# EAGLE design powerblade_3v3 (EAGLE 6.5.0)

## Sheet 1 of 6: AC-DC Power Supply
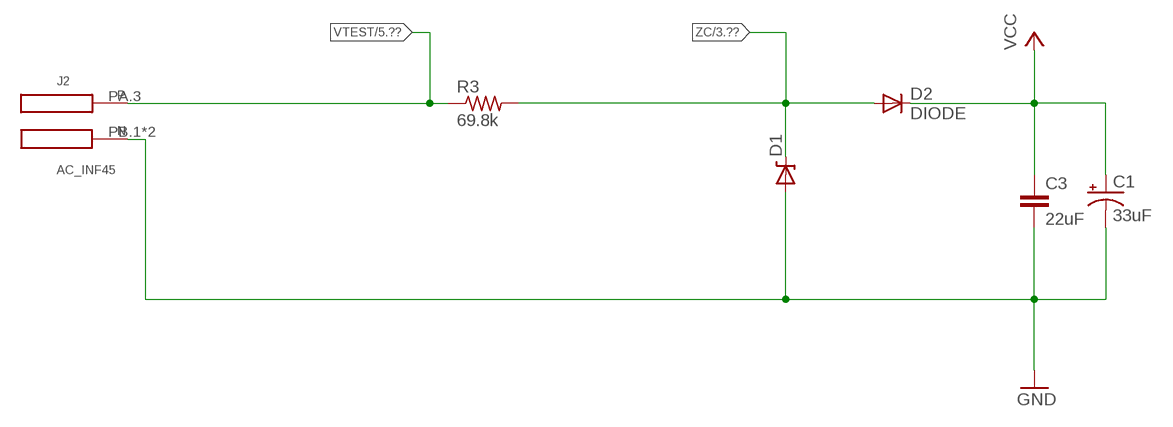
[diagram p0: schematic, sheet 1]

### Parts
C1  33uF  CPOL-US0805_SM  [CPOL0805_SM]
C3  22uF  C-EUC0603_SM  [C0603_SM]
D1  ZENERBZT52  [BZT52]
D2  DIODE  [BAS521]
J2  AC_INF45  [AC3_F45]
R3  69.8k  R-US_R1210  [R1210]

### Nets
GND: C1.- C3.2 D1.A J2.PB.1(N) J2.PB.3(N) ; also sheet 2,3,4,5,6
VCC: C1.+ C3.1 D2.C ; also sheet 2,3,6
VTEST: J2.PA.3(P) R3.1 ; also sheet 5
ZC: D1.C D2.A R3.2 ; also sheet 3,6

## Sheet 2 of 6: Load Supply Regulation
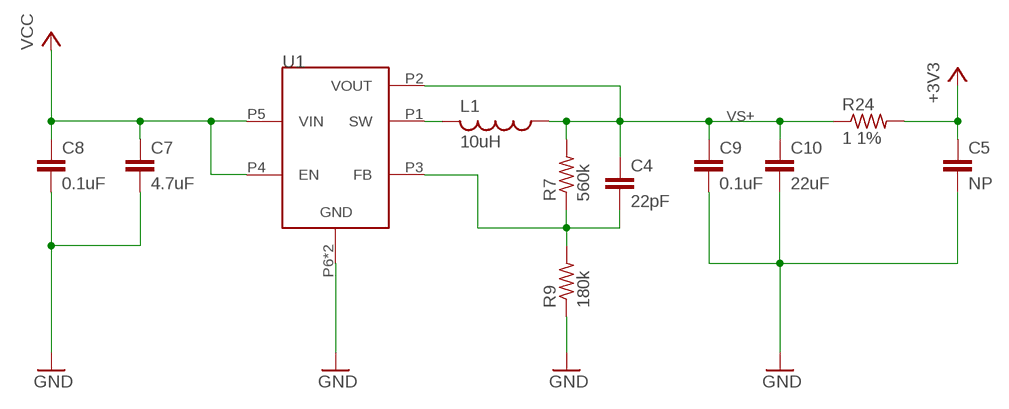
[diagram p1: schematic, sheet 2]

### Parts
C4  22pF  C-EUC0402  [C0402]
C5  NP  C-EUC0603_TN  [C0603_TN]
C7  4.7uF  C-EUC0402  [C0402]
C8  0.1uF  C-EUC0402  [C0402]
C9  0.1uF  C-EUC0402_SM  [C0402_SM]
C10  22uF  C-EUC0603_SM  [C0603_SM]
L1  10uH  L-USL0805  [L0805]
R7  560k  R-US_R0402  [R0402]
R9  180k  R-US_R0402  [R0402]
R24  1 1%  R-US_R0603_SM  [R0603_SM]
U1  TPS62122  [WDFN-6]

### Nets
+3V3: C5.1 R24.2 ; also sheet 3,4,5,6
GND: C5.2 C7.2 C8.2 C9.2 C10.2 R9.1 U1.P6(GND) U1.PAD(GND) ; also sheet 1,3,4,5,6
N$9: L1.2 U1.P1(SW)
N$13: C4.2 R7.1 R9.2 U1.P3(FB)
VCC: C7.1 C8.1 U1.P4(EN) U1.P5(VIN) ; also sheet 1,3,6
VS+: C4.1 C9.1 C10.1 L1.1 R7.2 R24.1 U1.P2(VOUT) ; also sheet 6

## Sheet 3 of 6: MSP430FR5738
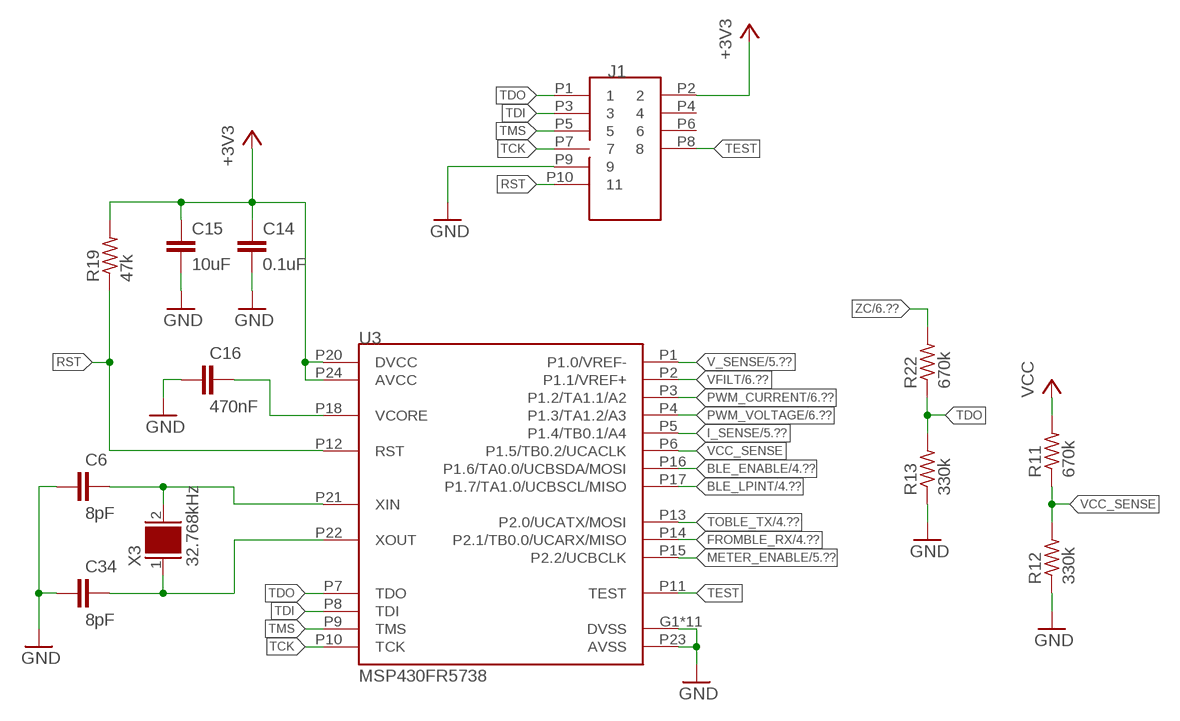
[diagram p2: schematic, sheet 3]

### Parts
C6  8pF  C-EUC0402  [C0402]
C14  0.1uF  C-EUC0402  [C0402]
C15  10uF  C-EUC0603_SM  [C0603_SM]
C16  470nF  C-EUC0402  [C0402]
C34  8pF  C-EUC0402  [C0402]
J1  JTAG_14PIN_IDC-ND  [TC2050-IDC-NL-430-ND]
R11  670k  R-US_R0402  [R0402]
R12  330k  R-US_R0402  [R0402]
R13  330k  R-US_R0402  [R0402]
R19  47k  R-US_R0402  [R0402]
R22  670k  R-US_R0402  [R0402]
U3  MSP430FR5738  [VQFN-24]
X3  32.768kHz  CRYSTAL_0805  [0805]

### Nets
+3V3: C14.1 C15.1 J1.P2 R19.2 U3.P20(DVCC) U3.P24(AVCC) ; also sheet 2,4,5,6
BLE_ENABLE: U3.P16(P1.6/TA0.0/UCBSDA/MOSI) ; also sheet 4
BLE_LPINT: U3.P17(P1.7/TA1.0/UCBSCL/MISO) ; also sheet 4
FROMBLE_RX: U3.P14(P2.1/TB0.0/UCARX/MISO) ; also sheet 4,6
GND: C6.1 C14.2 C15.2 C16.1 C34.1 J1.P9 R12.1 R13.1 U3.G1(DVSS) U3.G2(DVSS) U3.G3(DVSS) U3.G4(DVSS) U3.G5(DVSS) U3.G6(DVSS) U3.G7(DVSS) U3.G8(DVSS) U3.G9(DVSS) U3.P19(DVSS) U3.P23(AVSS) U3.PAD(DVSS) ; also sheet 1,2,4,5,6
I_SENSE: U3.P5(P1.4/TB0.1/A4) ; also sheet 5,6
METER_ENABLE: U3.P15(P2.2/UCBCLK) ; also sheet 5
N$3: C34.2 U3.P22(XOUT) X3.1
N$23: C16.2 U3.P18(VCORE)
N$56: C6.2 U3.P21(XIN) X3.2
PWM_CURRENT: U3.P3(P1.2/TA1.1/A2) ; also sheet 6
PWM_VOLTAGE: U3.P4(P1.3/TA1.2/A3) ; also sheet 6
RST: J1.P10 R19.1 U3.P12(RST)
TCK: J1.P7 U3.P10(TCK)
TDI: J1.P3 U3.P8(TDI)
TDO: J1.P1 R13.2 R22.1 U3.P7(TDO)
TEST: J1.P8 U3.P11(TEST)
TMS: J1.P5 U3.P9(TMS)
TOBLE_TX: U3.P13(P2.0/UCATX/MOSI) ; also sheet 4,6
V_SENSE: U3.P1(P1.0/VREF-) ; also sheet 5,6
VCC: R11.2 ; also sheet 1,2,6
VCC_SENSE: R11.1 R12.2 U3.P6(P1.5/TB0.2/UCACLK)
VFILT: U3.P2(P1.1/VREF+) ; also sheet 5,6
ZC: R22.2 ; also sheet 1,6
Unconnected: J1.P4 J1.P6

## Sheet 4 of 6: nr51822
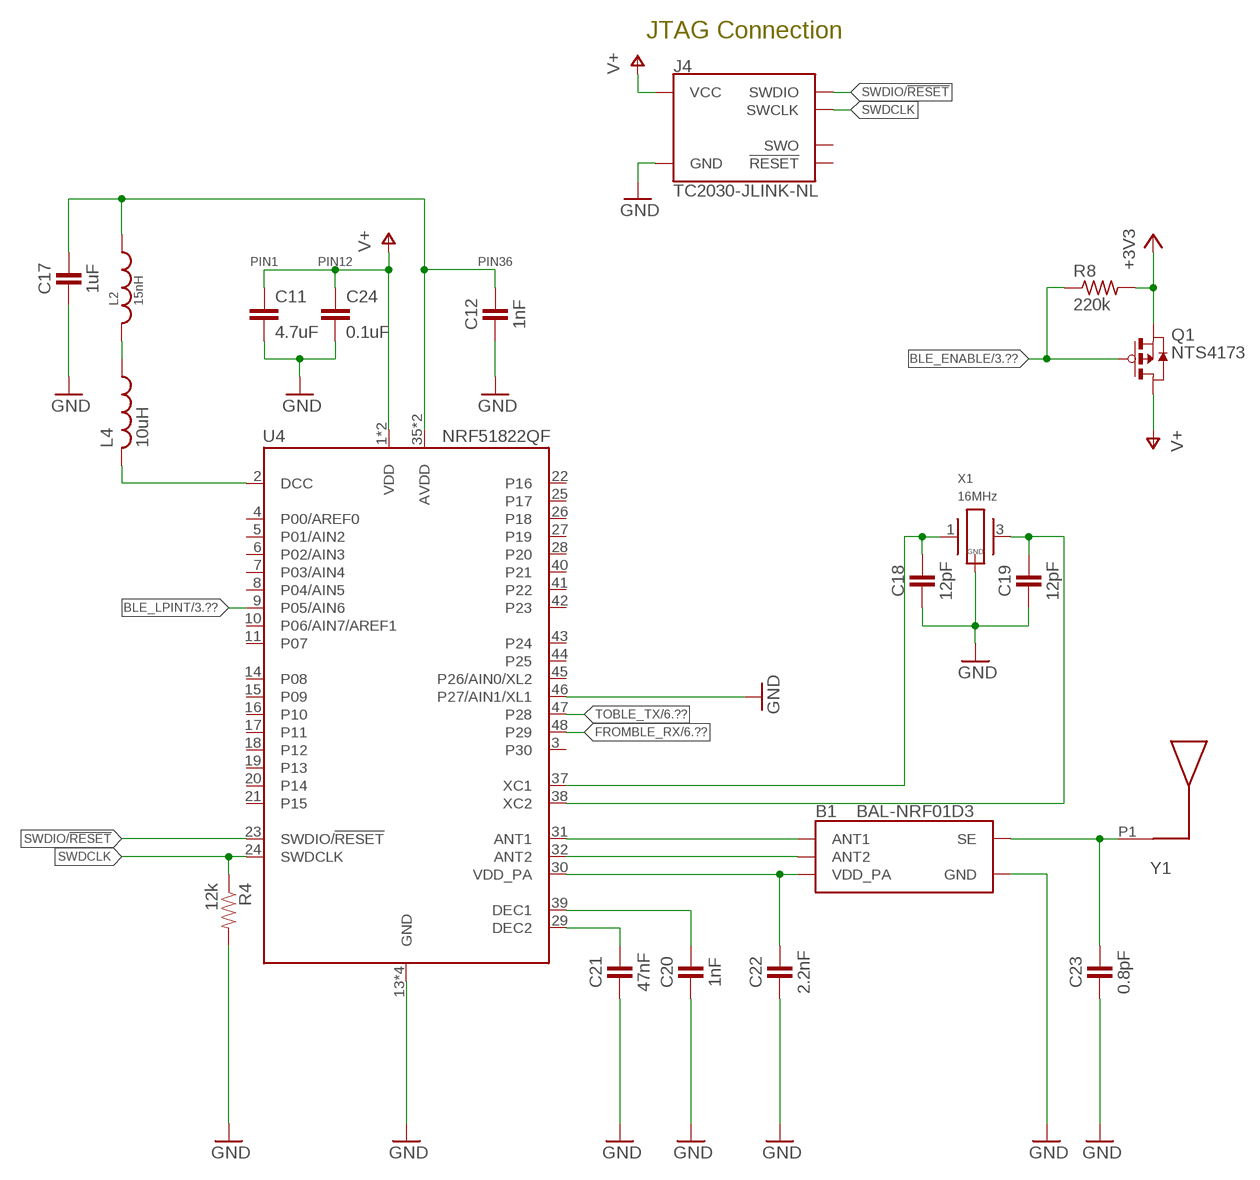
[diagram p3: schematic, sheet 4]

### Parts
B1  BAL-NRF01D3  [BAL-NRF01D3]
C11  4.7uF  C-EUC0402  [C0402]
C12  1nF  CAPACITOR  [0402_CAP]
C17  1uF  CAPACITOR  [0402_CAP]
C18  12pF  CAPACITOR  [0402_CAP]
C19  12pF  CAPACITOR  [0402_CAP]
C20  1nF  CAPACITOR  [0402_CAP]
C21  47nF  CAPACITOR  [0402_CAP]
C22  2.2nF  CAPACITOR  [0402_CAP]
C23  0.8pF  CAPACITOR  [0402_CAP]
C24  0.1uF  C-EUC0402  [C0402]
J4  TC2030-JLINK-NL  [TC2030-IDC-NL]
L2  15nH  INDUCTOR0402  [0402_CAP]
L4  10uH  L-USL0603_TN  [C0603_TN]
Q1  NTS4173  [SC-70-3]
R4  12k  RESISTOR  [0402_RES]
R8  220k  R-US_R0402_SM  [R0402_SM]
U4  NRF51822QF  [QFN-48-6MM]
X1  16MHz  TXC-8Y  [TXC-8Y]
Y1  UREACH_XTEND  [UREACH_XTEND]

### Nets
+3V3: Q1.P2(S) R8.2 ; also sheet 2,3,5,6
AVDD: C12.1 C17.1 L2.1 U4.35(AVDD) U4.36(AVDD)
BLE_ENABLE: Q1.P1(G) R8.1 ; also sheet 3
BLE_LPINT: U4.9(P05/AIN6) ; also sheet 3
DCC: L4.2 U4.2(DCC)
FROMBLE_RX: U4.48(P29) ; also sheet 3,6
GND: B1.GND C11.2 C12.2 C17.2 C18.2 C19.2 C20.2 C21.2 C22.2 C23.2 C24.2 J4.5(GND) R4.2 U4.13(GND) U4.33(GND) U4.34(GND) U4.46(P27/AIN1/XL1) U4.GND X1.2(GND) X1.4(GND) ; also sheet 1,2,3,5,6
N$4: B1.SE C23.1 Y1.P1
N$5: B1.ANT1 U4.31(ANT1)
N$6: B1.ANT2 U4.32(ANT2)
N$10: L2.2 L4.1
N$16: C18.1 U4.37(XC1) X1.1
N$17: C19.1 U4.38(XC2) X1.3
N$18: C20.1 U4.39(DEC1)
N$19: C21.1 U4.29(DEC2)
SWDCLK: J4.4(SWCLK) R4.1 U4.24(SWDCLK)
SWDIO/!RESET: J4.2(SWDIO) U4.23(SWDIO/!RESET)
TOBLE_TX: U4.47(P28) ; also sheet 3,6
V+: C11.1 C24.1 J4.1(VCC) Q1.P3(D) U4.1(VDD) U4.12(VDD)
VDD_PA: B1.VCC(VDD_PA) C22.1 U4.30(VDD_PA)
Unconnected: J4.3(!RESET) J4.6(SWO) U4.3(P30) U4.4(P00/AREF0) U4.5(P01/AIN2) U4.6(P02/AIN3) U4.7(P03/AIN4) U4.8(P04/AIN5) U4.10(P06/AIN7/AREF1) U4.11(P07) U4.14(P08) U4.15(P09) U4.16(P10) U4.17(P11) U4.18(P12) U4.19(P13) U4.20(P14) U4.21(P15) U4.22(P16) U4.25(P17) U4.26(P18) U4.27(P19) U4.28(P20) U4.40(P21) U4.41(P22) U4.42(P23) U4.43(P24) U4.44(P25) U4.45(P26/AIN0/XL2)

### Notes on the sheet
- JTAG Connection
- PIN1 | PIN12 | PIN36

## Sheet 5 of 6: Power Sensing!
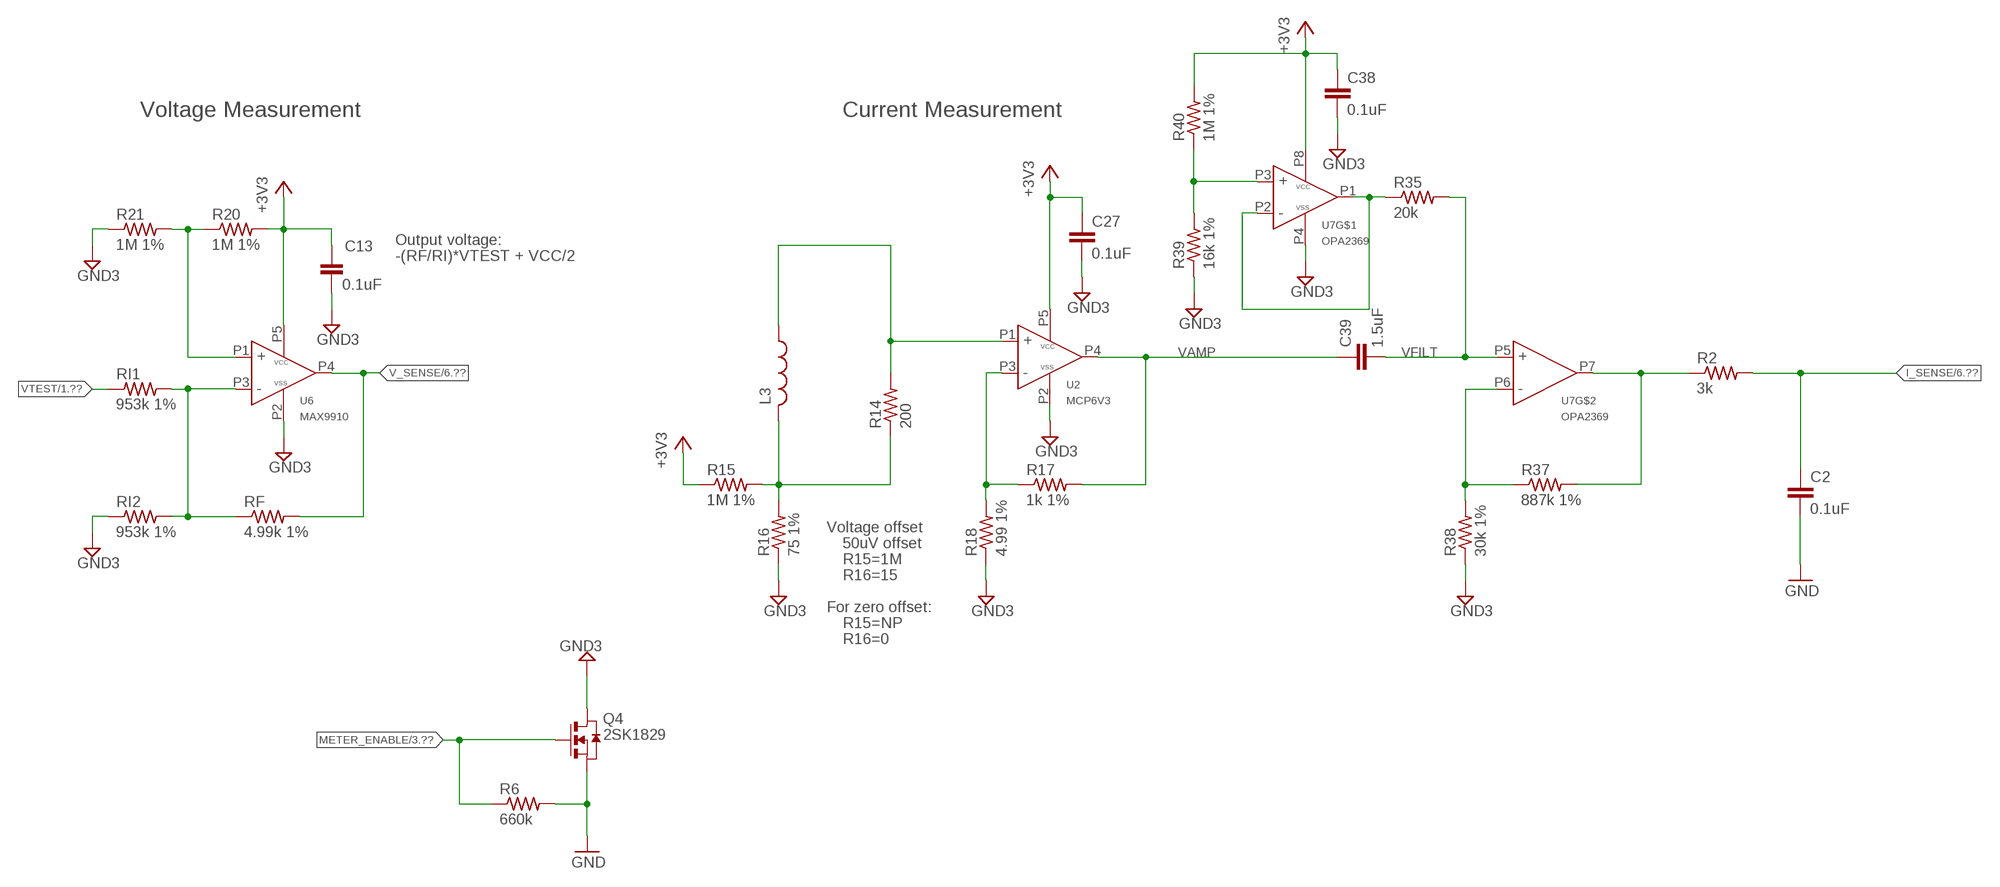
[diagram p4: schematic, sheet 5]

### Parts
C2  0.1uF  C-EUC0402  [C0402]
C13  0.1uF  CAPACITOR  [0402_CAP]
C27  0.1uF  C-EUC0402  [C0402]
C38  0.1uF  C-EUC0402  [C0402]
C39  1.5uF  C-EUC0402  [C0402]
L3  L-USL0805  [L0805]
Q4  2SK1829  [SC-70-3]
R2  3k  R-US_R0402_SM  [R0402_SM]
R6  660k  R-US_R0402  [R0402]
R14  200  R-US_R0402  [R0402]
R15  1M 1%  R-US_R0402  [R0402]
R16  75 1%  R-US_R0402  [R0402]
R17  1k 1%  R-US_R0402  [R0402]
R18  4.99 1%  R-US_R0402  [R0402]
R20  1M 1%  R-US_R0402  [R0402]
R21  1M 1%  R-US_R0402_SM  [R0402_SM]
R35  20k  R-US_R0402  [R0402]
R37  887k 1%  R-US_R0402  [R0402]
R38  30k 1%  R-US_R0402  [R0402]
R39  16k 1%  R-US_R0402  [R0402]
R40  1M 1%  R-US_R0402  [R0402]
RF  4.99k 1%  R-US_R0402  [R0402]
RI1  953k 1%  R-US_R0402  [R0402]
RI2  953k 1%  R-US_R0402  [R0402]
U2  MCP6V3  [SC70-5]
U6  MAX9910  [SC70-5]
U7  OPA2369  [SOT-23-8]

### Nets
+3V3: C13.1 C27.1 C38.1 R15.1 R20.2 R40.2 U2.P5(VCC) U6.P5(VCC) U7.P8(VCC) ; also sheet 2,3,4,6
GND: C2.2 Q4.P2(S) R6.2 ; also sheet 1,2,3,4,6
GND3: C13.2 C27.2 C38.2 Q4.P3(D) R16.1 R18.1 R21.1 R38.1 R39.1 RI2.1 U2.P2(VSS) U6.P2(VSS) U7.P4(VSS)
I_SENSE: C2.1 R2.2 ; also sheet 3,6
METER_ENABLE: Q4.P1(G) R6.1 ; also sheet 3
N$1: R2.1 R37.2 U7.P7(OUT)
N$37: L3.2 R14.1 R15.2 R16.2
N$38: L3.1 R14.2 U2.P1(IN+)
N$40: R20.1 R21.2 U6.P1(IN+)
N$41: RF.1 RI1.2 RI2.2 U6.P3(IN-)
N$65: R17.1 R18.2 U2.P3(IN-)
N$66: R37.1 R38.2 U7.P6(IN-)
N$68: R35.1 U7.P1(OUT) U7.P2(IN-)
N$70: R39.2 R40.1 U7.P3(IN+)
V_SENSE: RF.2 U6.P4(OUT) ; also sheet 3,6
VAMP: C39.1 R17.2 U2.P4(OUT)
VFILT: C39.2 R35.2 U7.P5(IN+) ; also sheet 3,6
VTEST: RI1.1 ; also sheet 1

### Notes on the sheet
- Voltage Measurement | Current Measurement
- Output voltage:
- -(RF/RI)*VTEST + VCC/2
- Voltage offset
- 50uV offset
- R15=1M
- R16=15
- For zero offset:
- R15=NP
- R16=0

## Sheet 6 of 6: Debugging Connector. OOF
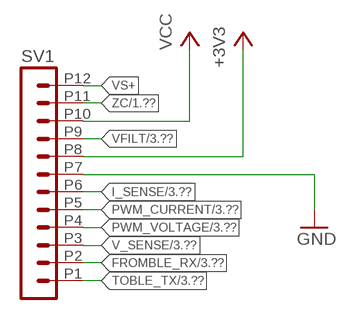
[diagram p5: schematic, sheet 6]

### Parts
SV1  MA12-11M27  [MA12-1_1MM27]

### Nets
+3V3: SV1.P8 ; also sheet 2,3,4,5
FROMBLE_RX: SV1.P2 ; also sheet 3,4
GND: SV1.P7 ; also sheet 1,2,3,4,5
I_SENSE: SV1.P6 ; also sheet 3,5
PWM_CURRENT: SV1.P5 ; also sheet 3
PWM_VOLTAGE: SV1.P4 ; also sheet 3
TOBLE_TX: SV1.P1 ; also sheet 3,4
V_SENSE: SV1.P3 ; also sheet 3,5
VCC: SV1.P10 ; also sheet 1,2,3
VFILT: SV1.P9 ; also sheet 3,5
VS+: SV1.P12 ; also sheet 2
ZC: SV1.P11 ; also sheet 1,3

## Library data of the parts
B1 = chips:BAL-NRF01D3: 50 ohm nominal input / conjugate match balun to nRF51422-QFAA, nRF24LE1, nRF51822-QFAA/AB, with integrated harmonic filter; DIGIKEY: 497-13637-1-ND; MOUSER: 511-BAL-NRF01D3
C1 = rcl:CPOL-US: POLARIZED CAPACITOR, American symbol; DIGIKEY: 478-8650-1-ND
C2 = rcl:C-EU: CAPACITOR, European symbol; DIGIKEY: 490-10777-1-ND
C3 C10 = rcl:C-EU: CAPACITOR, European symbol; DIGIKEY: 445-9077-1-ND
C4 = rcl:C-EU: CAPACITOR, European symbol; DIGIKEY: 445-1239-1-ND
C5 = rcl:C-EU: CAPACITOR, European symbol; DIGIKEY: NP
C6 C34 = rcl:C-EU: CAPACITOR, European symbol; DIGIKEY: 445-4890-1-ND
C7 = rcl:C-EU: CAPACITOR, European symbol; DIGIKEY: 445-8023-1-ND
C8 C9 C14 C24 C27 C38 = rcl:C-EU: CAPACITOR, European symbol; DIGIKEY: 445-4952-1-ND
C11 = rcl:C-EU: CAPACITOR, European symbol; DIGIKEY: 445-5947-1-ND
C12 C20 = passives:CAPACITOR: 0402 Capacitor; DIGIKEY: 490-1303-1-ND
C13 = passives:CAPACITOR: 0402 Capacitor; DIGIKEY: 445-4952-1-ND
C15 = rcl:C-EU: CAPACITOR, European symbol; DIGIKEY: 445-6853-1-ND
C16 = rcl:C-EU: CAPACITOR, European symbol; DIGIKEY: 445-4989-1-ND
C17 = passives:CAPACITOR: 0402 Capacitor; DIGIKEY: 1276-1513-1-ND
C18 C19 = passives:CAPACITOR: 0402 Capacitor; DIGIKEY: 490-6197-1-ND
C21 = passives:CAPACITOR: 0402 Capacitor; DIGIKEY: 445-1264-1-ND
C22 = passives:CAPACITOR: 0402 Capacitor; DIGIKEY: 490-5419-1-ND
C23 = passives:CAPACITOR: 0402 Capacitor; DIGIKEY: 490-6269-1-ND
C39 = rcl:C-EU: CAPACITOR, European symbol; DIGIKEY: 445-13815-1-ND
D1 = powerfilm:ZENER; DIGIKEY: BZT52C10T-7DICT-ND
D2 = powerfilm:DIODE; DIGIKEY: BAS521-7DICT-ND
J1 = ibat:JTAG_14PIN; DIGIKEY: NP
J2 = powerfilm:AC_IN; DIGIKEY: ED1649-ND; DIGIKEY_2: ED1649-ND; DIGIKEY_3: ED1649-ND; DIGIKEY_4: ED1649-ND
J4 = connector:TC2030-JLINK; DIGIKEY: NP
L1 = rcl:L-US: INDUCTOR, American symbol; DIGIKEY: 490-4990-1-ND
L2 = passives:INDUCTOR; DIGIKEY: 587-1521-1-ND
L3 = rcl:L-US: INDUCTOR, American symbol; DIGIKEY: 732-3452-1-ND
L4 = rcl:L-US: INDUCTOR, American symbol; DIGIKEY: 490-4025-1-ND
Q1 = powerfilm:NTS4173; DIGIKEY: NTS4173PT1GOSCT-ND
Q4 = powerfilm:2SK1829; DIGIKEY: 2SK1829TE85LFCT-ND
R2 = rcl:R-US_: RESISTOR, American symbol; DIGIKEY: P3.00KLCT-ND
R3 = rcl:R-US_: RESISTOR, American symbol; DIGIKEY: P69.8KAACT-ND
R4 = passives:RESISTOR: Resistor; DIGIKEY: RHM12.0KCDCT-ND
R6 R11 R22 = rcl:R-US_: RESISTOR, American symbol; DIGIKEY: P665KLCT-ND
R7 = rcl:R-US_: RESISTOR, American symbol; DIGIKEY: P560KLCT-ND
R8 = rcl:R-US_: RESISTOR, American symbol; DIGIKEY: P220KJCT-ND
R9 = rcl:R-US_: RESISTOR, American symbol; DIGIKEY: P180KLCT-ND
R12 R13 = rcl:R-US_: RESISTOR, American symbol; DIGIKEY: P330KLCT-ND
R14 = rcl:R-US_: RESISTOR, American symbol; DIGIKEY: P200LCT-ND
R15 R20 R21 R40 = rcl:R-US_: RESISTOR, American symbol; DIGIKEY: P1.00MLCT-ND
R16 = rcl:R-US_: RESISTOR, American symbol; DIGIKEY: P75.0LCT-ND
R17 = rcl:R-US_: RESISTOR, American symbol; DIGIKEY: P1.00KLCT-ND
R18 = rcl:R-US_: RESISTOR, American symbol; DIGIKEY: RMCF0402FT4R99CT-ND
R19 = rcl:R-US_: RESISTOR, American symbol; DIGIKEY: P47KJCT-ND
R24 = rcl:R-US_: RESISTOR, American symbol; DIGIKEY: P1.0AJCT-ND
R35 = rcl:R-US_: RESISTOR, American symbol; DIGIKEY: P20.0KLCT-ND
R37 = rcl:R-US_: RESISTOR, American symbol; DIGIKEY: P887KLCT-ND
R38 = rcl:R-US_: RESISTOR, American symbol; DIGIKEY: P30.0KLCT-ND
R39 = rcl:R-US_: RESISTOR, American symbol; DIGIKEY: P16.0KLCT-ND
RF = rcl:R-US_: RESISTOR, American symbol; DIGIKEY: P4.99KLCT-ND
RI1 RI2 = rcl:R-US_: RESISTOR, American symbol; DIGIKEY: P953KLCT-ND
SV1 = con-lstb:MA12-1: PIN HEADER; DIGIKEY: S9014E-12-ND
U1 = powerfilm:TPS62122; DIGIKEY: 296-27695-1-ND
U2 = powerfilm:MCP6V3; DIGIKEY: 296-19547-1-ND
U3 = powerfilm:MSP430FR5738; DIGIKEY: 296-29232-1-ND
U4 = chips:NRF51822: Multiprotocol Bluetooth® 4.0 low energy/2.4 GHz RF SoC; DIGIKEY: 1490-1032-1-ND; MOUSER: 949-NRF51822-QFAB-R7
U6 = powerfilm:MAX9910; DIGIKEY: 296-25252-1-ND
U7 = powerfilm:OPA2369; DIGIKEY: 296-22671-1-ND
X1 = crystals:TXC-8Y: 2mmx1.6mm SMD Crystal; DIGIKEY: 887-2003-1-ND
X3 = general:CRYSTAL_0805; DIGIKEY: 535-12373-1-ND
Y1 = powerfilm:UREACH_XTEND; FRACTUS: FR05-S1-N-0-110

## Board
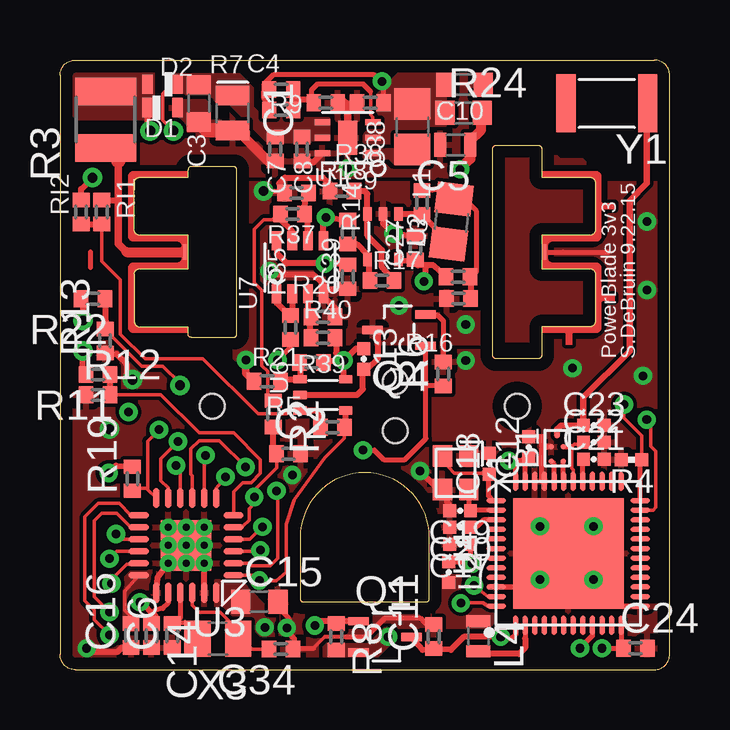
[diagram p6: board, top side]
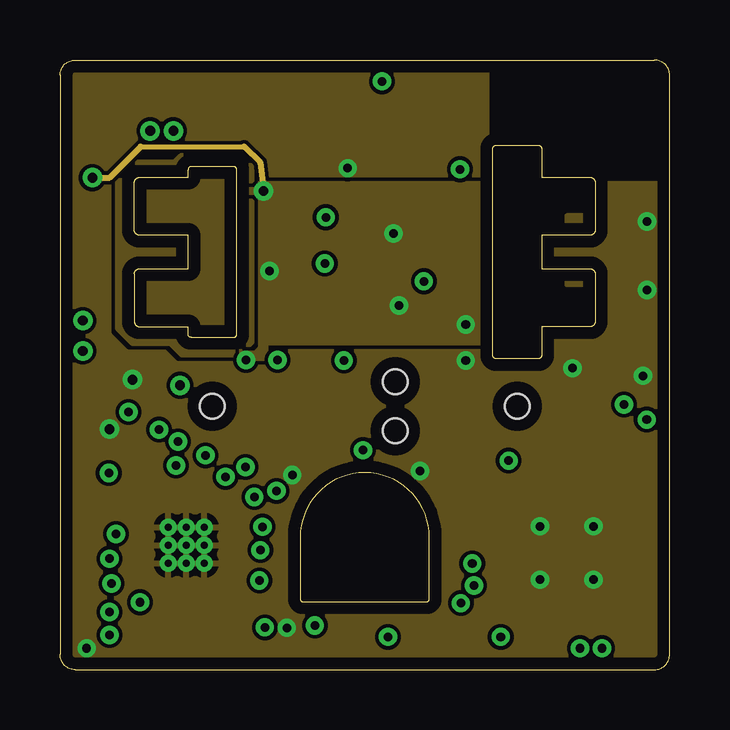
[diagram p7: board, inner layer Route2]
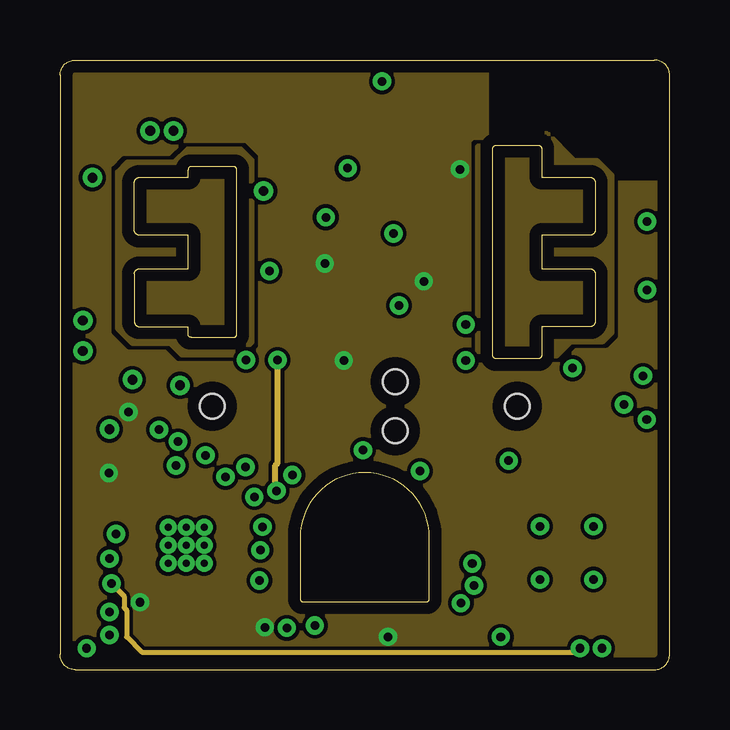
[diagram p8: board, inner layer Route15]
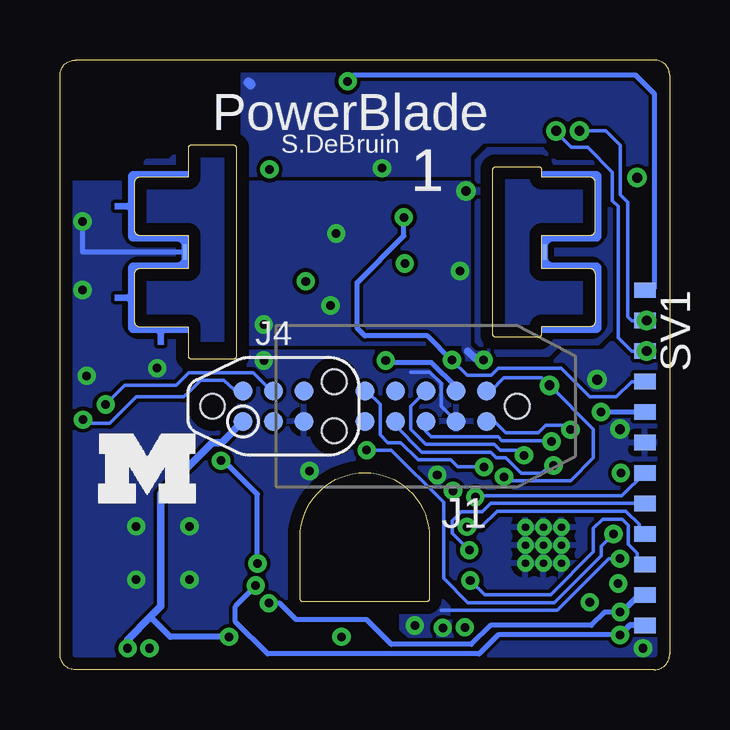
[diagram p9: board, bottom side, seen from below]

Size 25.4 x 25.4 mm. Coordinates in mm from the lower left corner, seen from the top.
Copper layers (1+2*15+16): Top 0.0178mm / dielectric 12mil / Route2 0.0356mm / dielectric 28mil / Route15 0.0356mm / dielectric 12mil / Bottom 0.0178mm
Design rules "SSC-EAGLE-4Lyr_v1.0.0.3 *": minimum track width 6mil, minimum drill 8mil, track to track 6mil, track to pad 6mil, pad to pad 6mil, via to via 6mil, smd to smd 6mil, copper to edge 20mil, drill to drill 16mil, minimum pad ring 8mil, minimum via ring 8mil, stop-mask expansion 3mil, vias tented up to drill 0mil, thermal gap 10mil

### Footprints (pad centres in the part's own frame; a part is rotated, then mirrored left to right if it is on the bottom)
BAL-NRF01D3 = smd 0.22 x 0.22: ANT1 -0.537,-0.25; ANT2 -0.537,0.25; GND 0.069,0.25; SE 0.537,0; VCC 0.069,-0.25
CPOL0805_SM = smd 0.8 x 1.4: + -0.73,0; - 0.73,0
C0402 = smd 0.6 x 0.7: 1 -0.5,0; 2 0.5,0
C0603_SM = smd 0.8 x 1: 1 -0.775,0; 2 0.775,0
C0603_TN = smd 0.5 x 1: 1 -0.625,0; 2 0.625,0
C0402_SM = smd 0.6 x 0.7: 1 -0.55,0; 2 0.55,0
0402_CAP = smd 0.536 x 0.546: 1 -0.433,0; 2 0.433,0
BZT52 = smd 0.45 x 0.8: A -0.625,0; C 0.625,0
BAS521 = smd 0.45 x 0.8: A -0.625,0; C 0.625,0
TC2050-IDC-NL-430-ND = smd 0.787 x 0.787: P1 -2.54,-0.635; P2 -1.27,-0.635; P3 0,-0.635; P4 1.27,-0.635; P5 2.54,-0.635; P6 2.54,0.635; P7 1.27,0.635; P8 0,0.635; P9 -1.27,0.635; P10 -2.54,0.635 | hole 1.029: -3.81,0
AC3_F45 = smd 0.152 x 0.635 bottom: PA.1 -7.493,0; PB.1 7.493,0 | smd 0.152 x 0.635: PA.3 -7.493,0; PB.3 7.493,0
TC2030-IDC-NL = smd 0.787 x 0.787: 1 -1.27,-0.635; 2 -1.27,0.635; 3 0,-0.635; 4 0,0.635; 5 1.27,-0.635; 6 1.27,0.635 | hole 1.016: -2.54,0; 2.54,1.016; 2.54,-1.016
L0805 = smd 1.3 x 1.5: 1 -0.95,0; 2 0.95,0
SC-70-3 = smd 0.85 x 0.35: P1 -1.1,0.65; P2 -1.1,-0.65; P3 1.1,0
R0402_SM = smd 0.6 x 0.7: 1 -0.55,0; 2 0.55,0
R1210 = smd 1.15 x 2.55: 1 -1.175,0; 2 1.175,0
0402_RES = smd 0.536 x 0.546: 1 -0.433,0; 2 0.433,0
R0402 = smd 0.6 x 0.7: 1 -0.5,0; 2 0.5,0
R0603_SM = smd 0.8 x 1: 1 -0.775,0; 2 0.775,0
MA12-1_1MM27 = smd 0.889 x 0.635: P1 0,6.985; P2 0,5.715; P3 0,4.445; P4 0,3.175; P5 0,1.905; P6 0,0.635; P7 0,-0.635; P8 0,-1.905; P9 0,-3.175; P10 0,-4.445; P11 0,-5.715; P12 0,-6.985
WDFN-6 = smd 0.65 x 0.25: P1 -1.05,0.65; P2 -1.05,0; P3 -1.05,-0.65; P4 1.05,-0.65; P5 1.05,0; P6 1.05,0.65 | smd 0.8 x 1.4: PAD 0,0
SC70-5 = smd 0.55 x 0.35: P1 -0.95,0.65; P2 -0.95,0; P3 -0.95,-0.65; P4 0.95,-0.65; P5 0.95,0.65
VQFN-24 = drill 0.3 pad 0.5: G1 -0.75,0.75; G2 0,0.75; G3 0.75,0.75; G4 -0.75,0; G5 0,0; G6 0.75,0; G7 -0.75,-0.75; G8 0,-0.75; G9 0.75,-0.75 | smd 0.85 x 0.28: P1 -1.975,1.25; P2 -1.975,0.75; P3 -1.975,0.25; P4 -1.975,-0.25; P5 -1.975,-0.75; P6 -1.975,-1.25; P13 1.975,-1.25; P14 1.975,-0.75; P15 1.975,-0.25; P16 1.975,0.25; P17 1.975,0.75; P18 1.975,1.25 | smd 0.28 x 0.85: P7 -1.25,-1.975; P8 -0.75,-1.975; P9 -0.25,-1.975; P10 0.25,-1.975; P11 0.75,-1.975; P12 1.25,-1.975; P19 1.25,1.975; P20 0.75,1.975; P21 0.25,1.975; P22 -0.25,1.975; P23 -0.75,1.975; P24 -1.25,1.975 | smd 2.1 x 2.1: PAD 0,0
QFN-48-6MM = smd 0.8 x 0.203: 1 -3,2.2; 2 -3,1.8; 3 -3,1.4; 4 -3,1; 5 -3,0.6; 6 -3,0.2; 7 -3,-0.2; 8 -3,-0.6; 9 -3,-1; 10 -3,-1.4; 11 -3,-1.8; 12 -3,-2.2; 25 3,-2.2; 26 3,-1.8; 27 3,-1.4; 28 3,-1; 29 3,-0.6; 30 3,-0.2; 31 3,0.2; 32 3,0.6; 33 3,1; 34 3,1.4; 35 3,1.8; 36 3,2.2 | smd 0.203 x 0.8: 13 -2.2,-3; 14 -1.8,-3; 15 -1.4,-3; 16 -1,-3; 17 -0.6,-3; 18 -0.2,-3; 19 0.2,-3; 20 0.6,-3; 21 1,-3; 22 1.4,-3; 23 1.8,-3; 24 2.2,-3; 37 2.2,3; 38 1.8,3; 39 1.4,3; 40 1,3; 41 0.6,3; 42 0.2,3; 43 -0.2,3; 44 -0.6,3; 45 -1,3; 46 -1.4,3; 47 -1.8,3; 48 -2.2,3 | smd 4.6 x 4.6: GND 0,0
SOT-23-8 = smd 0.8 x 0.4: P1 -1.1,0.975; P2 -1.1,0.325; P3 -1.1,-0.325; P4 -1.1,-0.975; P5 1.1,-0.975; P6 1.1,-0.325; P7 1.1,0.325; P8 1.1,0.975
TXC-8Y = smd 0.9 x 0.8: 1 -0.7,-0.55; 2 0.7,-0.55; 3 0.7,0.55; 4 -0.7,0.55
0805 = smd 1.1 x 1.5: 1 -0.85,0; 2 0.85,0
UREACH_XTEND = smd 0.8 x 2.4: NC 1.7,0; P1 -1.7,0

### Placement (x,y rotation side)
B1  20.72,9.22 90 top
C1  7.19,23.19 270 top
C2  9.52,8.99 0 top
C3  5.79,23.59 270 top
C4  9.22,23.32 0 top
C5  16.48,21.86 180 top
C6  4.67,1.41 90 top
C7  8.97,21.69 270 top
C8  10.08,21.69 270 top
C9  12.93,23.62 180 top
C10  16.86,24.37 0 top
C11  15.57,1.37 90 top
C12  19.53,9.27 90 top
C13  12.65,12.94 270 top
C14  3.81,1.41 270 top
C15  8.31,2.82 0 top
C16  2.96,1.42 90 top
C17  16.67,5.23 180 top
C18  17.88,8.58 90 top
C19  16.67,6.62 180 top
C20  16.67,5.92 180 top
C21  22.24,8.76 0 top
C22  22.24,9.47 0 top
C23  22.24,10.18 0 top
C24  23.98,0.89 0 top
C27  14.81,17.58 90 top
C34  9.2,0.86 180 top
C38  11.99,16.37 270 top
C39  11.99,18.24 90 top
D1  4.27,23.42 180 top
D2  4.27,24.38 0 top
J1  10.16,10.97 180 bottom
J2  12.7,17.4 0 top
J4  16.51,10.97 0 bottom
L1  14.68,22.62 270 top
L2  16.19,4.06 270 top
L3  16.31,18.67 82.9 top
L4  17.43,1.4 270 top
Q1  13.54,1.37 0 top
Q4  14.13,14.14 180 top
R2  8.89,10.65 270 top
R3  1.9,22.91 90 top
R4  23.81,8.75 180 top
R6  15.97,12.32 90 top
R7  9.22,24.17 180 top
R8  11.51,1.37 270 top
R9  11.07,23.62 180 top
R11  1.59,12.3 180 top
R12  1.59,11.45 0 top
R13  1.88,13.7 90 top
R14  15.08,19.46 270 top
R15  16.59,16.37 0 top
R16  16.61,15.46 0 top
R17  13.41,16.21 180 top
R18  11.75,19.94 0 top
R19  3.02,7.95 90 top
R20  10.48,12.8 0 top
R21  8.64,12.01 0 top
R22  1.38,15.46 180 top
R24  16.81,23.19 0 top
R35  9.6,14.25 270 top
R37  9.68,18.99 180 top
R38  9.86,19.86 0 top
R39  10.95,14.7 180 top
R40  10.95,13.83 0 top
RF  11.35,10.1 0 top
RI1  1.74,19.07 270 top
RI2  0.88,19.07 270 top
SV1  1.03,8.83 180 bottom
U1  11.99,22.16 180 top
U2  13.46,18.03 270 top
U3  5.25,5.18 180 top
U4  21.18,4.84 90 top
U6  10.95,11.45 0 top
U7  10,16.76 90 top
U$1  [BLOCK-M]  23.81,6.92 0 bottom
X1  16.48,8.2 270 top
X3  6.58,1.28 180 top
Y1  22.78,23.6 180 top

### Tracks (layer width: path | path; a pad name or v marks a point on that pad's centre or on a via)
+3V3  (via drill 0.36)
  Top 0.203: U3.P20 4.5,2.77 4.29,2.56 3.97,2.48 3.85,2.36
  Top 0.254: R15.1 15.56,16.84 15.16,16.84 | U2.P5 14.17,17.03 C27.1 14.81,16.96 14.92,16.84 15.16,16.84 | v15.16,16.18 15.24,16.26 15.24,16.76 15.16,16.84 | C38.1 11.98,16.92 v11.03,16.92 9.45,16.92 9.05,17.32 9.05,17.84 U7.P8 | C14.1 3.97,2.24 3.85,2.36 3.48,2.73 v3.33,2.81 | R40.2 11.51,13.82 11.51,13.2 v11.83,12.88 | v2.03,8.19 2.34,8.5 R19.2 | R20.2 11.06,12.88 v11.83,12.88 | v11.83,12.88 12.32,13.37 C13.1 | U6.P5 11.83,12.17 v11.83,12.88
  Top 0.406: v16.67,20.85 17.1,21.28 C5.1 17.1,22.04 17.54,22.48 17.54,23.15 R24.2
  Bottom 0.203: SV1.P8 v2.86,10.73 | J1.P2 8.89,11.76 9.92,12.8 11.74,12.8 v11.83,12.88
  other vias: 8.53,1.76 13.67,1.37
  pour Route15 (rank 2): -0.32,-0.38 24.89,-0.38 24.89,20.26 17.78,20.26 17.78,26.29 -0.32,26.29
  pour Top (no thermals): 6.51,2.32 7.54,2.32 8.49,1.37 8.97,1.37 9.13,1.52 9.13,1.92 7.54,3.67 6.51,3.67
  pour Top (no thermals): 11.03,0.57 13.18,0.57 13.65,1.05 13.65,1.6 13.41,1.84 12.46,1.84 11.67,1.05 11.03,1.05
AVDD  (via drill 0.36)
  Top 0.203: U4.35 19.38,8.7 19.44,8.75 | 19.44,8.75 C12.1 | 19.44,8.75 19.37,8.83 19.25,8.71 19.05,8.71 | L2.1 17.1,4.5 v17.18,4.42 17.1,4.5 C17.1 | 19.05,8.71 v18.69,8.71 | U4.36 18.98,8.64 19.05,8.71
  Bottom 0.203: v17.18,4.42 17.18,7.31 18.57,8.71 v18.69,8.71
BLE_ENABLE  (via drill 0.36)
  Top 0.152: U3.P16 2.37,4.93 v2.06,4.62
  Top 0.254: Q1.P1 11.45,2.02 | 11.45,2.02 R8.1 | 11.45,2.02 10.79,2.02 v10.62,1.84
  Bottom 0.152: 9.52,2.48 4.68,2.48 2.54,4.62 v2.06,4.62
  pour Bottom (no thermals): 9.21,2.64 9.21,1.6 9.45,1.37 10.87,1.37 11.19,1.68 11.19,2.71 10.79,3.11 9.68,3.11
BLE_LPINT  (via drill 0.36)
  Top 0.152: U3.P17 2.98,4.43 2.94,4.38 2.78,4.38 2.14,3.75 v2.14,3.59
  Top 0.203: U4.9 22.18,1.4 v21.67,0.89
  Route15 0.203: v2.14,3.59 2.67,3.06 2.67,2.58 2.78,2.48 2.78,1.37 3.41,0.73 21.51,0.73 v21.67,0.89
DCC
  Top 0.203: U4.2 19.38,1.3
  Top 0.254: 19.38,1.3 19.38,0.91 19.13,0.65 17.74,0.65 L4.2
FROMBLE_RX  (via drill 0.36)
  Top 0.152: U4.48 17.85,2.64 17.62,2.79 16.73,2.79 v16.7,2.77 | v2.06,2.4 1.43,3.03 1.43,6.21 1.75,6.53 2.36,6.53 2.96,5.93 U3.P14
  Bottom 0.203: v2.06,2.4 2.7,2.4 3.25,1.84 7.46,1.84 8.25,1.05 11.59,1.05 12.62,2.08 15.56,2.08 16.25,2.77 v16.7,2.77
  Bottom 0.254: SV1.P2 1.27,3.11 1.9,2.48 1.98,2.48 v2.06,2.4
GND  (via drill 0.36, 0.41)
  Top 0.152: 10.56,0.89 11.03,1.37 11.91,1.37
  Top 0.203: C15.2 9.08,2.6 9.52,2.16 9.52,1.52 9.76,1.29 9.76,0.81 9.84,0.89 10.56,0.89 | C19.2 16.24,6.88 16.11,7 16.11,7.32 X1.2 | U4.13 21.18,2.64 21.18,4.06 | 21.18,4.06 U4.GND | U4.33 20.08,7.84 20.08,9.22 20.15,9.29 B1.GND 20.46,9.3 20.08,9.3 20.08,9.7 C12.2 | U4.46 20.56,3.44 21.07,3.95 21.18,4.06 | 11.91,1.37 12.75,1.37 13.55,2.16 15,2.16 15.24,1.92 C11.2 15.54,1.92 | Q4.P2 15.24,14.78 15.72,14.78 15.97,14.53 R6.2 | 20.95,17.4 J2.PB.1 22.86,17.4
  Top 0.254: U3.P19 4.07,3.85 U3.G3 | U1.P6 10.56,21.14 C8.2 | U3.P23 U3.G1 | X1.2 15.77,7.5 v15,8.27 | v20,3.75 20.87,3.75 21.07,3.95 | R13.1 2.35,13.15 2.78,12.72 2.78,12.32 v3.02,12.08 | C16.1 2.57,0.92 2.38,0.73 1.27,0.73 v1.11,0.89
  Top 0.305: U1.PAD 11.99,23.51 11.75,23.75 R9.1
  Top 0.406: C1.- 7.2,22.48 7.62,22.48 7.7,22.4 7.7,22.16 8.68,21.19 C7.2
  Top 0.61: C3.2 6.14,22.46 C1.-
  Bottom 0.152: J1.P9 9.52,10.97 9.52,11.92 10,12.4 10.79,12.4
  Bottom 0.203: J2.PB.1 24.46,17.4 v24.46,18.67
  Bottom 0.406: 17.54,24.46 17.46,24.38
  other vias: 9.45,1.74 21.35,12.56 16.91,12.87 11.99,20.89 24.29,12.24 22.23,3.75 20,5.97 22.23,5.97 24.46,15.81 2.06,10.02 9.68,8.11
  pour Top (rank 6): -1.27,26.54 17.78,26.54 17.78,20.27 24.89,20.27 24.89,-0.38 -1.27,-0.38
  pour Bottom (rank 6): -1.27,26.54 17.78,26.54 17.78,20.27 24.89,20.27 24.89,-0.38 -1.27,-0.38
  pour Route2 (rank 6): -1.27,26.54 4.13,26.54 4.13,26.53 17.78,26.54 17.78,20.27 24.89,20.27 24.89,-0.38 -1.27,-0.38
  pour Route2 (no thermals): 21.11,18.91 21.11,16.05 22.7,16.05 22.7,16.13 22.7,18.91
  pour Top (no thermals): 4.76,22.96 5.24,22.48 6.19,22.48 6.19,23.51 6.03,23.67 4.76,23.67
GND3  (via drill 0.36, 0.41)
  Top 0.203: v8.48,19.94 9.28,19.94 R38.1
  Top 0.254: C27.2 13.94,18.13 v13.89,18.17 13.46,18.6 U2.P2 | R38.1 9.13,20.26 9.37,20.5 10.95,20.5 11.19,20.26 11.19,19.95 R18.1 | U7.P4 10.98,15.55 11.51,15.02 11.51,14.71 R39.1 | C38.2 11.13,15.82 U7.P4 | U7.P4 10.98,16.11 10.56,16.45 8.89,16.45 v8.73,16.61 | U6.P2 12.38,11.45 12.62,11.68 12.62,12.48 C13.2 12.81,12.51 13.26,12.95 13.26,14.08 Q4.P3 | RI2.1 0.88,20.03 v1.35,20.5
  Top 0.305: v7.75,12.9 7.75,12.35 R21.1
  Route2 0.203: 3.36,21.79 7.67,21.79
  Route2 0.254: v1.35,20.5 2.06,20.5 3.36,21.79 | 7.67,21.79 8.33,21.13 v8.48,19.94
  Bottom 0.305: v7.75,12.9 8.04,12.9 8.41,13.27
  other vias: 14.13,15.18 16.91,14.38
  pour Bottom (rank 4): 18.1,13.59 8.57,13.59 8.57,12.95 7.3,12.95 7.3,20.26 18.1,20.26
  pour Route2 (rank 4): 18.1,13.59 8.57,13.59 8.57,12.95 7.3,12.95 7.3,20.26 18.1,20.26
  pour Top (rank 4): 18.1,13.59 8.57,13.59 8.57,12.95 7.3,12.95 7.3,20.26 18.1,20.26
I_SENSE  (via drill 0.36)
  Top 0.152: U3.P5 7.27,5.97 7.62,5.97 7.88,6.23 7.88,6.71 8.1,6.92 v8.1,7.19 8.1,7.48 9.02,8.41 C2.1
  Top 0.254: C2.1 8.89,9.13 R2.2
  Bottom 0.152: SV1.P6 1.98,7.24 8.04,7.24 v8.1,7.19
METER_ENABLE  (via drill 0.36)
  Top 0.152: U3.P15 2.61,5.43 v2.34,5.65
  Top 0.203: v12.62,9.14 13.1,9.14 13.49,8.75 14.37,8.75 15.24,9.62 15.24,11.82 | Q4.P1 15.24,13.48 15.24,12 15.24,11.82 | R6.1 15.24,11.82
  Bottom 0.152: 2.38,5.65 v2.34,5.65 2.86,5.13 2.86,4.75 4.82,2.79 8.41,2.79 9.42,3.8 9.42,6.98 11.59,9.14 v12.62,9.14
N$1
  Top 0.152: 8.92,18.77 8.9,18.75 8.49,18.75 8.1,18.35 8.1,16.13 8.41,15.81 8.41,12.66 8.65,12.42 8.65,11.44 R2.1
  Top 0.203: 8.97,18.99 R37.2 8.92,18.77
  Top 0.254: U7.P7 9.68,18.28 9.21,18.75 9.21,18.91 R37.2
N$3
  Top 0.152: C34.2 8.02,0.86 X3.1 7.3,1.58 7.3,1.76 6.67,2.4 5.79,2.4 5.5,2.69 U3.P22
N$4
  Top 0.254: B1.SE 20.72,10.02 20.88,10.18 C23.1
  Top 0.267: C23.1 21.81,11.35 23.73,13.27 23.73,19.54 24.45,20.26 24.45,23.56
  Top 0.381: 24.45,23.56 Y1.P1
N$5
  Top 0.203: U4.31 20.97,7.86 B1.ANT1
N$6
  Top 0.203: U4.32 20.58,8.57 B1.ANT2
N$9
  pour Top (rank 3, no thermals): 12.7,21.37 13.73,21.37 13.97,21.13 15.32,21.13 15.32,22.24 14.21,22.24 13.57,21.61 12.7,21.61
N$10
  pour Top (rank 2, no thermals): 15.8,1.76 17.86,1.76 18.1,2 18.1,2.95 16.67,3.11 16.67,3.91 15.72,3.91 15.64,3.83 15.64,1.92
N$13
  Top 0.152: U1.P3 13.04,23.02 12.94,23.11 12.94,24.08
  Top 0.203: 12.94,24.08 12.62,24.41 10.74,24.41 10.48,24.15 10.48,23.75
  Top 0.254: R7.1 9.68,23.75 | 9.68,23.75 C4.2 | 9.68,23.75 10.48,23.75 R9.2
N$16
  Top 0.152: 17.62,8.19 16.43,8.19 16.19,8.43 16.19,8.64 X1.1
  Top 0.203: U4.37 18.06,7.04 17.86,7.24 17.86,8.12 C18.1 17.67,8.15 17.62,8.19
N$17
  Top 0.203: U4.38 17.12,6.64 | 17.12,6.64 C19.1 | X1.3 17.04,6.73 17.12,6.64
N$18
  Top 0.203: U4.39 17.66,6.24 17.38,5.97 17.15,5.97 C20.1
N$19
  Top 0.203: U4.29 21.78,8.73 C21.1
N$23
  Top 0.152: U3.P18 2.7,3.27 2.7,2.48 3.09,2.09 C16.2
  pour Top (rank 2, no thermals): 3.81,4.06 3.02,4.06 2.7,3.75 2.7,1.68 3.49,1.68 3.49,2.32 3.81,2.64
N$37
  Top 0.203: R15.2 17.36,16.59 17.36,19.09 16.83,19.62 16.51,19.62 16.5,19.61 L3.2
  Top 0.254: L3.2 16.02,20.01 R14.1 15.01,19.94 | R15.2 17.14,15.5 17.14,15.49 17.14,15.47 R16.2
N$38
  Top 0.254: L3.1 16.19,17.8 R14.2 15.01,18.98 U2.P1
N$40
  Top 0.254: R20.1 10,12.77 U6.P1 9.27,12.1 R21.2
N$41
  Top 0.152: RI1.2 1.74,17.01 2.51,16.23 2.51,13.98 3.54,12.95 5.95,12.95 8.25,10.65 9.45,10.65 9.59,10.8 U6.P3
  Top 0.254: U6.P3 10.65,10.8 10.85,10.6 RF.1 | RI2.2 RI1.2
N$56
  Top 0.203: 4.84,2.08 4.84,1.98 C6.2 | C6.2 5.22,1.96 X3.2 | U3.P21 5,2.14 C6.2
N$65
  Top 0.254: R18.2 12.7,19.94 12.81,19.83 U2.P3 12.81,18.08 13.41,17.48 13.41,16.76 R17.1
N$66
  Top 0.254: U7.P6 10.33,18.89 R37.1 10.23,19.76 R38.2
N$68
  Top 0.254: R35.1 9.49,14.82 | 9.49,14.82 9.03,15.28 U7.P1 | U7.P2 9.68,15.01 9.49,14.82
N$70
  Top 0.254: U7.P3 10.33,14.78 R39.2 10.48,14.77 | R40.1 10.4,14.47 10.48,14.54 10.48,14.77 | 10.48,14.86 10.48,14.77
PWM_CURRENT  (via drill 0.36)
  Top 0.152: U3.P3 8.3,4.93 v8.35,4.98
  Bottom 0.152: SV1.P5 7.46,6.92 7.8,6.58 8.68,6.58 9.05,6.21 9.05,5.68 v8.35,4.98
PWM_VOLTAGE  (via drill 0.36)
  Top 0.152: U3.P4 7.91,5.43 v8.44,5.95
  Bottom 0.152: SV1.P4 1.27,5.65 1.27,6.05 1.83,6.6 7.19,6.6 7.84,5.95 v8.44,5.95
RST  (via drill 0.36)
  Top 0.152: 3.65,7.56 3.65,9.52 v4.13,10 | 3.65,7.56 3.65,7.55 3.64,7.56 3.17,7.56 3.02,7.4 R19.1 | U3.P12 3.65,7.5 3.65,7.56
  Bottom 0.152: J1.P10 7.31,10.34 6.83,9.86 5.48,9.86 5.16,10.18 4.3,10.18 v4.13,10
SWDCLK  (via drill 0.36)
  Top 0.152: R4.1 24.25,9.74 23.49,10.49 v23.49,11.05
  Top 0.203: U4.24 24.18,8.69 R4.1
  Bottom 0.152: J4.4 16.64,11.65 17.36,12.37 20.03,12.37 20.56,11.84 22.7,11.84 v23.49,11.05
SWDIO/!RESET  (via drill 0.36)
  Top 0.152: U4.23 24.72,6.64 24.82,6.76 24.82,9.09 24.61,9.3 24.61,10.26 v24.45,10.41
  Bottom 0.152: J4.2 18.14,11.65 18.57,12.07 19.53,12.07 20,11.61 20.24,11.37 22.23,11.37 23.34,10.26 24.29,10.26 v24.45,10.41
TCK  (via drill 0.36)
  Top 0.152: U3.P10 5,8.35 4.96,8.4 v4.84,8.51
  Bottom 0.152: J1.P7 11.43,10.18 10.32,9.07 7.46,9.07 7.22,8.83 6.83,8.83 6.19,8.19 5.32,8.19 5,8.51 v4.84,8.51
TDI  (via drill 0.36)
  Top 0.152: U3.P8 6,8.79 v6.06,8.93
  Bottom 0.152: J1.P3 10.79,10.97 10.79,10.02 10.16,9.38 7.3,9.38 7.06,9.14 6.36,9.14 v6.06,8.93
TDO  (via drill 0.36, 0.41)
  Top 0.152: U3.P7 6.5,7.55 v6.9,8.03 | R13.2 2.14,13.98 2.14,13.91 3.41,12.64 4.29,12.64 5,11.92 v5,11.84
  Top 0.254: R13.2 1.93,14.3 R22.1
  Bottom 0.152: J1.P1 7.46,11.61 6.91,12.16 5.32,12.16 v5,11.84 3.17,10.02 3.17,8.83 4.13,7.87 6.83,7.87 v6.9,8.03
TEMP
  Top 0.203: 1.27,17.4 1.27,16.76
  pour Route15: 4.76,21.13 2.78,21.13 2.38,20.73 2.38,14.22 3.02,13.59 4.6,13.59 5.08,13.11 7.46,13.11 8.02,13.67 8.02,21.21 7.54,21.69 5.32,21.69
  pour Route15: 21.27,13.67 22.62,13.67 23.02,14.07 23.02,20.57 22.38,21.21 21.43,21.21 20.32,22.32 17.94,22.32 17.38,21.76 17.38,12.95 17.86,12.48 20.08,12.48
  pour Bottom: 4.76,21.13 2.78,21.13 2.38,20.73 2.38,14.22 3.02,13.59 4.6,13.59 5.08,13.11 7.46,13.11 8.02,13.67 8.02,21.21 7.54,21.69 5.32,21.69
  pour Top: 4.76,21.13 2.78,21.13 2.38,20.73 2.38,14.22 3.02,13.59 4.6,13.59 5.08,13.11 7.46,13.11 8.02,13.67 8.02,21.21 7.54,21.69 5.32,21.69
  pour Route2: 4.76,21.13 2.78,21.13 2.38,20.73 2.38,14.22 3.02,13.59 4.6,13.59 5.08,13.11 7.46,13.11 8.02,13.67 8.02,21.21 7.54,21.69 5.32,21.69
  pour Top: 20.64,14.3 21.99,14.3 22.38,14.7 22.38,20.57 21.75,21.21 20.8,21.21 20.32,21.69 18.57,21.69 18.02,21.13 18.02,14.22 18.49,13.75 20.08,13.75
  pour Bottom: 20.64,14.3 21.99,14.3 22.38,14.7 22.38,20.57 21.75,21.21 20.8,21.21 20.32,21.69 18.57,21.69 18.02,21.13 18.02,14.22 18.49,13.75 20.08,13.75
TEST  (via drill 0.36)
  Top 0.152: U3.P11 4.5,7.58 4.21,7.87 4.21,8.78 v4.91,9.5
  Bottom 0.152: J1.P8 10.16,9.94 9.92,9.7 7.14,9.7 6.98,9.54 5.05,9.54 v4.91,9.5
TMS  (via drill 0.36)
  Top 0.152: U3.P9 5.5,8.08 5.45,8.14 5.45,9.2 5.79,9.54 6.64,9.54 v7.73,8.45
  Bottom 0.152: J1.P5 12.62,11.61 12.06,11.05 12.06,9.78 11.75,9.46 11.19,9.46 10.48,8.75 9.13,8.75 8.83,8.45 v7.73,8.45
TOBLE_TX  (via drill 0.36)
  Top 0.152: v2.06,1.45 1.43,2.08 1.43,2.48 1.03,2.87 1.03,6.37 1.59,6.92 2.46,6.92 2.96,6.43 U3.P13 | U4.47 17.85,3.04 17.22,3.51
  Top 0.203: U3.P13 3.41,6.44 | 17.22,3.51 v17.25,3.51
  Bottom 0.203: v2.06,1.45 7.14,1.45 7.94,0.65 16.75,0.65 18.1,2 18.1,2.64 17.25,3.49 v17.25,3.51
  Bottom 0.254: SV1.P1 1.67,1.84 v2.06,1.45
V+  (via drill 0.36)
  Top 0.203: U4.12 23.38,0.98 C24.1 v22.58,0.89 | U4.1 18.98,1.46 18.81,1.29 18.44,1.29 v18.36,1.37
  Top 0.254: v18.36,1.37 16.83,1.37 16.28,0.82 C11.1 15.11,0.82 Q1.P3
  Bottom 0.254: v18.36,1.37 20.8,1.37 21.63,2.2
  Bottom 0.305: J4.1 18.66,9.46 19.05,9.46 21.19,7.32 21.19,2.64 21.63,2.2 22.58,1.25 v22.58,0.89
V_SENSE  (via drill 0.36)
  Top 0.152: RF.2 11.85,9.64 11.03,8.83 9.76,7.08 9.42,6.05 9.42,4.06 9.01,3.71 v8.31,3.71 8.09,3.93 U3.P1
  Top 0.254: RF.2 11.9,10.15 U6.P4
  Bottom 0.152: 1.27,4.38 1.35,4.46 1.35,4.86 1.72,5.23 1.72,6.02 1.97,6.27 2.79,6.27 3.17,5.89 3.17,4.91 4.95,3.11 7.7,3.11 v8.31,3.71
  Bottom 0.203: SV1.P3 1.27,4.38
VAMP
  Top 0.254: C39.1 12.02,17.72 12.38,17.72 12.81,17.29 U2.P4 12.86,17.03 R17.2
VCC  (via drill 0.41)
  Top 0.152: D2.C 4.68,24.38 4.29,23.99 4.29,22.89 v4.72,22.45
  Top 0.254: R11.2 0.95,12.44 v0.95,13.27
  Bottom 0.152: SV1.P10 1.59,13.27 2.14,13.83 2.14,19.3 2.38,19.54 2.38,20.73 3.41,21.77 4.1,21.77 4.72,22.38 v4.72,22.45
  Bottom 0.203: 1.27,13.27 SV1.P10
  Bottom 0.254: SV1.P10 v0.95,13.27
  pour Top (rank 2, no thermals): 11.19,22.08 10.48,22.08 10.4,22 8.65,22 7.06,23.59 6.59,23.59 6.19,23.99 4.68,23.99 4.68,24.78 7.46,24.78 8.02,24.23 8.02,23.43 8.49,22.96 11.19,22.96
VCC_SENSE
  Top 0.152: R12.2 4.21,11.45 5.79,9.86 7.23,9.86 8.34,8.75 8.34,8.18 7.96,7.8 7.62,7.8 7.23,7.4 U3.P6
  Top 0.254: R12.2 R11.1
VDD_PA
  Top 0.152: U4.30 21.38,8.32 21.31,8.39 21.31,9.27 21.43,9.38 21.73,9.38 C22.1
  Top 0.203: B1.VCC 21.29,9.29 21.31,9.27
VFILT  (via drill 0.36)
  Top 0.152: 9.09,12.88 v9.07,12.9 | v9.02,7.45 9.07,7.42 9.07,4.65 8.76,4.33 7.99,4.33 7.89,4.43 U3.P2
  Top 0.203: R35.2 9.6,13.43 v9.07,12.9
  Top 0.254: U7.P5 10.98,18.75 v11.07,18.85 11.13,18.79 C39.2
  Route15 0.254: v9.02,7.45 8.97,7.5 8.97,8.51 9.07,8.61 v9.07,12.9
  Bottom 0.152: v9.07,12.9 8.44,12.27 7.43,12.27 7.14,12.56 4.52,12.56 3.33,11.37 2.22,11.37 1.59,12 SV1.P9
  Bottom 0.203: v9.07,12.9 10.08,13.91 12.7,13.91 13.02,14.22 13.02,16.13 11.07,18.07 v11.07,18.85
VS+  (via drill 0.36)
  Top 0.203: C9.1 13.49,24.39 13.41,24.46 | 13.41,24.46 13.1,24.78 8.89,24.78 8.49,24.38 8.49,24.07 | 13.41,24.46 v13.41,24.51
  Top 0.254: C4.1 8.57,23.2 8.57,23.75 8.49,23.83 8.49,24.07 R7.2
  Bottom 0.203: v13.41,24.51 13.14,24.78 1.43,24.78 0.63,23.99 0.63,15.89 1.03,15.73 SV1.P12
  pour Top (rank 2, no thermals): 12.7,22 14.6,22 15.32,22.72 16.03,22.72 16.03,24.78 14.13,24.78 13.26,23.91 13.26,22.8 12.7,22.24
VTEST
  Top 0.152: 5.08,17.4 J2.PA.3
  Top 0.254: RI1.1 2.38,19.57 2.43,19.62
  Top 0.305: 2.43,21.2 2.43,19.62 2.43,17.74 2.78,17.4
  Top 0.406: R3.1 2.43,21.2 | 2.78,17.4 5.08,17.4
  Top 0.61: 2.43,21.21 2.43,21.2
ZC  (via drill 0.41)
  Top 0.254: R22.2 0.95,15.46 v0.95,14.54 | D1.C 3.64,22.57 v3.76,22.45
  Bottom 0.152: SV1.P11 1.59,14.54 1.75,14.7 1.75,19.46 2.06,19.78 2.06,21.84 2.67,22.45 v3.76,22.45
  Bottom 0.254: SV1.P11 v0.95,14.54
  pour Top (no thermals): 3.89,22.96 0.71,22.96 0.56,23.11 0.56,24.86 3.89,24.86

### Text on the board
tPlace: PowerBlade 3v3 | S.DeBruin 9.22.15
bPlace: PowerBlade | S.DeBruin

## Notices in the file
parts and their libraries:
SparkFun-Aesthetics: Licensing: CC v3.0 Share-Alike You are welcome to use this library for commercial purposes.
